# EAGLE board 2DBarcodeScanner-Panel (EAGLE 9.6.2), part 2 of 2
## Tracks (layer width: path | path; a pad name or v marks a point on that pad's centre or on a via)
3.3V  (via drill 0.38)
  Top 0.203: J4.3 23.37,16.38 29.34,22.35 32.3,22.35 J3.11 32.37,22.35 v34.04,22.35 | R7.2 43.14,24.64 v41.02,24.64 40.98,24.68 Q2.3 | 25.59,23.21 C2.1 | U1.5 25.59,23.21 | 25.59,23.21 25.59,22.41 v24.64,21.46
  Bottom 0.203: v24.64,21.46 25.53,22.35 v34.04,22.35 38.73,22.35 v41.02,24.64 | PWR.2 17.02,25.53 16.38,24.89 13.08,24.89 12.19,24 12.19,14.1 15.37,10.92 22.61,10.92 23.37,10.16 J4.3
3.3V1  (via drill 0.38)
  Top 0.203: J5.3 70.87,16.38 76.83,22.35 79.8,22.35 J6.11 79.87,22.35 v81.53,22.35 | R12.2 90.64,24.64 v88.52,24.64 88.48,24.68 Q4.3 | 73.09,23.21 C5.1 | U4.5 73.09,23.21 | 73.09,23.21 73.09,22.41 v72.14,21.46
  Bottom 0.203: v72.14,21.46 73.03,22.35 v81.53,22.35 86.23,22.35 v88.52,24.64 | PWR1.2 64.52,25.53 63.88,24.89 60.58,24.89 59.69,24 59.69,14.1 62.86,10.92 70.1,10.92 70.87,10.16 J5.3
3.3V2  (via drill 0.38)
  Top 0.203: J8.3 23.37,42.29 29.34,48.26 32.3,48.26 J9.11 32.37,48.26 v34.04,48.26 | R21.2 43.14,50.55 v41.02,50.55 40.98,50.59 Q6.3 | 25.59,49.12 C8.1 | U6.5 25.59,49.12 | 25.59,49.12 25.59,48.32 v24.64,47.37
  Bottom 0.203: v24.64,47.37 25.53,48.26 v34.04,48.26 38.73,48.26 v41.02,50.55 | PWR2.2 17.02,51.43 16.38,50.8 13.08,50.8 12.19,49.91 12.19,40 15.37,36.83 22.61,36.83 23.37,36.07 J8.3
3.3V3  (via drill 0.38)
  Top 0.203: J11.3 70.87,42.29 76.83,48.26 79.8,48.26 J12.11 79.87,48.26 v81.53,48.26 | R30.2 90.64,50.55 v88.52,50.55 88.48,50.59 Q8.3 | 73.09,49.12 C11.1 | U8.5 73.09,49.12 | 73.09,49.12 73.09,48.32 v72.14,47.37
  Bottom 0.203: v72.14,47.37 73.03,48.26 v81.53,48.26 86.23,48.26 v88.52,50.55 | PWR3.2 64.52,51.43 63.88,50.8 60.58,50.8 59.69,49.91 59.69,40 62.86,36.83 70.1,36.83 70.87,36.07 J11.3
3.3V4  (via drill 0.38)
  Top 0.203: J14.3 23.37,68.2 29.34,74.17 32.3,74.17 J15.11 32.37,74.17 v34.04,74.17 | R39.2 43.14,76.45 v41.02,76.45 40.98,76.5 Q10.3 | 25.59,75.03 C14.1 | U10.5 25.59,75.03 | 25.59,75.03 25.59,74.23 v24.64,73.28
  Bottom 0.203: v24.64,73.28 25.53,74.17 v34.04,74.17 38.73,74.17 v41.02,76.45 | PWR4.2 17.02,77.34 16.38,76.71 13.08,76.71 12.19,75.82 12.19,65.91 15.37,62.74 22.61,62.74 23.37,61.98 J14.3
3.3V5  (via drill 0.38)
  Top 0.203: J17.3 70.87,68.2 76.83,74.17 79.8,74.17 J18.11 79.87,74.17 v81.53,74.17 | R48.2 90.64,76.45 v88.52,76.45 88.48,76.5 Q12.3 | 73.09,75.03 C17.1 | U12.5 73.09,75.03 | 73.09,75.03 73.09,74.23 v72.14,73.28
  Bottom 0.203: v72.14,73.28 73.03,74.17 v81.53,74.17 86.23,74.17 v88.52,76.45 | PWR5.2 64.52,77.34 63.88,76.71 60.58,76.71 59.69,75.82 59.69,65.91 62.86,62.74 70.1,62.74 70.87,61.98 J17.3
3.3V6  (via drill 0.38)
  Top 0.203: J20.3 23.37,94.11 29.34,100.08 32.3,100.08 J21.11 32.37,100.08 v34.04,100.08 | R57.2 43.14,102.36 v41.02,102.36 40.98,102.41 Q14.3 | 25.59,100.94 C20.1 | U14.5 25.59,100.94 | 25.59,100.94 25.59,100.14 v24.64,99.19
  Bottom 0.203: v24.64,99.19 25.53,100.08 v34.04,100.08 38.73,100.08 v41.02,102.36 | PWR6.2 17.02,103.25 16.38,102.62 13.08,102.62 12.19,101.73 12.19,91.82 15.37,88.65 22.61,88.65 23.37,87.88 J20.3
3.3V7  (via drill 0.38)
  Top 0.203: J23.3 70.87,94.11 76.83,100.08 79.8,100.08 J24.11 79.87,100.08 v81.53,100.08 | R66.2 90.64,102.36 v88.52,102.36 88.48,102.41 Q16.3 | 73.09,100.94 C23.1 | U16.5 73.09,100.94 | 73.09,100.94 73.09,100.14 v72.14,99.19
  Bottom 0.203: v72.14,99.19 73.03,100.08 v81.53,100.08 86.23,100.08 v88.52,102.36 | PWR7.2 64.52,103.25 63.88,102.62 60.58,102.62 59.69,101.73 59.69,91.82 62.86,88.65 70.1,88.65 70.87,87.88 J23.3
5V  (via drill 0.38)
  Top 0.178: 25.62,27.3 U1.1
  Top 0.203: J2.VBUS1 15.5,22.1 v17.02,22.1 | v17.02,17.02 15.5,17.02 J2.VBUS2 | v25.53,30.1 25.49,30.06 C1.1 25.62,28.83 25.62,27.3 25.62,26.25 25.27,25.91 24,25.91 23.69,26.22 U1.3
  Bottom 0.203: v17.02,22.1 v17.02,17.02 20.83,17.02 23.37,19.56 23.37,27.94 v25.53,30.1
5V1  (via drill 0.38)
  Top 0.178: 73.12,27.3 U4.1
  Top 0.203: J1.VBUS1 63,22.1 v64.52,22.1 | v64.52,17.02 63,17.02 J1.VBUS2 | v73.03,30.1 72.99,30.06 C4.1 73.12,28.83 73.12,27.3 73.12,26.25 72.77,25.91 71.5,25.91 71.19,26.22 U4.3
  Bottom 0.203: v64.52,22.1 v64.52,17.02 68.33,17.02 70.87,19.56 70.87,27.94 v73.03,30.1
5V2  (via drill 0.38)
  Top 0.178: 25.62,53.21 U6.1
  Top 0.203: J7.VBUS1 15.5,48.01 v17.02,48.01 | v17.02,42.93 15.5,42.93 J7.VBUS2 | v25.53,56.01 25.49,55.97 C7.1 25.62,54.73 25.62,53.21 25.62,52.16 25.27,51.82 24,51.82 23.69,52.13 U6.3
  Bottom 0.203: v17.02,48.01 v17.02,42.93 20.83,42.93 23.37,45.47 23.37,53.85 v25.53,56.01
5V3  (via drill 0.38)
  Top 0.178: 73.12,53.21 U8.1
  Top 0.203: J10.VBUS1 63,48.01 v64.52,48.01 | v64.52,42.93 63,42.93 J10.VBUS2 | v73.03,56.01 72.99,55.97 C10.1 73.12,54.73 73.12,53.21 73.12,52.16 72.77,51.82 71.5,51.82 71.19,52.13 U8.3
  Bottom 0.203: v64.52,48.01 v64.52,42.93 68.33,42.93 70.87,45.47 70.87,53.85 v73.03,56.01
5V4  (via drill 0.38)
  Top 0.178: 25.62,79.12 U10.1
  Top 0.203: J13.VBUS1 15.5,73.91 v17.02,73.91 | v17.02,68.83 15.5,68.83 J13.VBUS2 | v25.53,81.92 25.49,81.88 C13.1 25.62,80.64 25.62,79.12 25.62,78.07 25.27,77.72 24,77.72 23.69,78.04 U10.3
  Bottom 0.203: v17.02,73.91 v17.02,68.83 20.83,68.83 23.37,71.37 23.37,79.76 v25.53,81.92
5V5  (via drill 0.38)
  Top 0.178: 73.12,79.12 U12.1
  Top 0.203: J16.VBUS1 63,73.91 v64.52,73.91 | v64.52,68.83 63,68.83 J16.VBUS2 | v73.03,81.92 72.99,81.88 C16.1 73.12,80.64 73.12,79.12 73.12,78.07 72.77,77.72 71.5,77.72 71.19,78.04 U12.3
  Bottom 0.203: v64.52,73.91 v64.52,68.83 68.33,68.83 70.87,71.37 70.87,79.76 v73.03,81.92
5V6  (via drill 0.38)
  Top 0.178: 25.62,105.03 U14.1
  Top 0.203: J19.VBUS1 15.5,99.82 v17.02,99.82 | v17.02,94.74 15.5,94.74 J19.VBUS2 | v25.53,107.82 25.49,107.78 C19.1 25.62,106.55 25.62,105.03 25.62,103.98 25.27,103.63 24,103.63 23.69,103.95 U14.3
  Bottom 0.203: v17.02,99.82 v17.02,94.74 20.83,94.74 23.37,97.28 23.37,105.66 v25.53,107.82
5V7  (via drill 0.38)
  Top 0.178: 73.12,105.03 U16.1
  Top 0.203: J22.VBUS1 63,99.82 v64.52,99.82 | v64.52,94.74 63,94.74 J22.VBUS2 | v73.03,107.82 72.99,107.78 C22.1 73.12,106.55 73.12,105.03 73.12,103.98 72.77,103.63 71.5,103.63 71.19,103.95 U16.3
  Bottom 0.203: v64.52,99.82 v64.52,94.74 68.33,94.74 70.87,97.28 70.87,105.66 v73.03,107.82
!SCAN_TRIGGER!  (via drill 0.38)
  Top 0.203: v35.31,24.64 S2.3 35.31,20.95 25.91,11.56 J4.2 | C3.1 35.27,27.43 v35.31,27.39 J3.1
  Bottom 0.203: v35.31,24.64 v35.31,27.39
!SCAN_TRIGGER!1  (via drill 0.38)
  Top 0.203: v82.8,24.64 S1.3 82.8,20.95 73.41,11.56 J5.2 | C6.1 82.77,27.43 v82.8,27.39 J6.1
  Bottom 0.203: v82.8,24.64 v82.8,27.39
!SCAN_TRIGGER!2  (via drill 0.38)
  Top 0.203: v35.31,50.55 S3.3 35.31,46.86 25.91,37.46 J8.2 | C9.1 35.27,53.33 v35.31,53.3 J9.1
  Bottom 0.203: v35.31,50.55 v35.31,53.3
!SCAN_TRIGGER!3  (via drill 0.38)
  Top 0.203: v82.8,50.55 S4.3 82.8,46.86 73.41,37.46 J11.2 | C12.1 82.77,53.33 v82.8,53.3 J12.1
  Bottom 0.203: v82.8,50.55 v82.8,53.3
!SCAN_TRIGGER!4  (via drill 0.38)
  Top 0.203: v35.31,76.45 S5.3 35.31,72.77 25.91,63.37 J14.2 | C15.1 35.27,79.24 v35.31,79.2 J15.1
  Bottom 0.203: v35.31,76.45 v35.31,79.2
!SCAN_TRIGGER!5  (via drill 0.38)
  Top 0.203: v82.8,76.45 S6.3 82.8,72.77 73.41,63.37 J17.2 | C18.1 82.77,79.24 v82.8,79.2 J18.1
  Bottom 0.203: v82.8,76.45 v82.8,79.2
!SCAN_TRIGGER!6  (via drill 0.38)
  Top 0.203: v35.31,102.36 S7.3 35.31,98.68 25.91,89.28 J20.2 | C21.1 35.27,105.15 v35.31,105.11 J21.1
  Bottom 0.203: v35.31,102.36 v35.31,105.11
!SCAN_TRIGGER!7  (via drill 0.38)
  Top 0.203: v82.8,102.36 S8.3 82.8,98.68 73.41,89.28 J23.2 | C24.1 82.77,105.15 v82.8,105.11 J24.1
  Bottom 0.203: v82.8,102.36 v82.8,105.11
BUZZER  (via drill 0.38)
  Top 0.203: v41.15,29.59 R9.1 | J3.4 31.01,25.89 v30.99,25.91
  Bottom 0.203: v30.99,25.91 30.99,28.45 32.13,29.59 v41.15,29.59
BUZZER1  (via drill 0.38)
  Top 0.203: v88.65,29.59 R14.1 | J6.4 78.51,25.89 v78.49,25.91
  Bottom 0.203: v78.49,25.91 78.49,28.45 79.63,29.59 v88.65,29.59
BUZZER2  (via drill 0.38)
  Top 0.203: v41.15,55.5 R23.1 | J9.4 31.01,51.8 v30.99,51.82
  Bottom 0.203: v30.99,51.82 30.99,54.36 32.13,55.5 v41.15,55.5
BUZZER3  (via drill 0.38)
  Top 0.203: v88.65,55.5 R32.1 | J12.4 78.51,51.8 v78.49,51.82
  Bottom 0.203: v78.49,51.82 78.49,54.36 79.63,55.5 v88.65,55.5
BUZZER4  (via drill 0.38)
  Top 0.203: v41.15,81.41 R41.1 | J15.4 31.01,77.7 v30.99,77.72
  Bottom 0.203: v30.99,77.72 30.99,80.26 32.13,81.41 v41.15,81.41
BUZZER5  (via drill 0.38)
  Top 0.203: v88.65,81.41 R50.1 | J18.4 78.51,77.7 v78.49,77.72
  Bottom 0.203: v78.49,77.72 78.49,80.26 79.63,81.41 v88.65,81.41
BUZZER6  (via drill 0.38)
  Top 0.203: v41.15,107.31 R59.1 | J21.4 31.01,103.61 v30.99,103.63
  Bottom 0.203: v30.99,103.63 30.99,106.17 32.13,107.31 v41.15,107.31
BUZZER7  (via drill 0.38)
  Top 0.203: v88.65,107.31 R68.1 | J24.4 78.51,103.61 v78.49,103.63
  Bottom 0.203: v78.49,103.63 78.49,106.17 79.63,107.31 v88.65,107.31
CC1
  Top 0.178: J1.A5 63.19,20.81
  Top 0.203: 63.19,20.81 65.85,20.81 R6.2
CC2
  Top 0.203: J1.B5 66.23,17.81 R5.2
CC3
  Top 0.178: J2.A5 15.69,20.81
  Top 0.203: 15.69,20.81 18.36,20.81 R3.2
CC4
  Top 0.203: J2.B5 18.74,17.81 R2.2
CC5
  Top 0.178: J7.A5 15.69,46.72
  Top 0.203: 15.69,46.72 18.36,46.72 R20.2
CC6
  Top 0.203: J7.B5 18.74,43.72 R19.2
CC7
  Top 0.178: J10.A5 63.19,46.72
  Top 0.203: 63.19,46.72 65.85,46.72 R29.2
CC8
  Top 0.203: J10.B5 66.23,43.72 R28.2
CC9
  Top 0.178: J13.A5 15.69,72.62
  Top 0.203: 15.69,72.62 18.36,72.62 R38.2
CC10
  Top 0.203: J13.B5 18.74,69.62 R37.2
CC11
  Top 0.178: J16.A5 63.19,72.62
  Top 0.203: 63.19,72.62 65.85,72.62 R47.2
CC12
  Top 0.203: J16.B5 66.23,69.62 R46.2
CC13
  Top 0.178: J19.A5 15.69,98.53
  Top 0.203: 15.69,98.53 18.36,98.53 R56.2
CC14
  Top 0.203: J19.B5 18.74,95.53 R55.2
CC15
  Top 0.178: J22.A5 63.19,98.53
  Top 0.203: 63.19,98.53 65.85,98.53 R65.2
CC16
  Top 0.203: J22.B5 66.23,95.53 R64.2
GND  (via drill 0.38)  (25 unrouted)
  Top 0.203: C1.2 24.64,28.11 U1.2 | C2.2 24.64,23.96 v24.64,24.64 | J3.10 33.43,22.89 v34.04,23.5
  other vias: 14.48,25.91 13.21,25.91 19.56,24.64 10.67,20.83 10.67,18.29 28.57,20.19 34.04,24.64 28.45,28.45 28.45,27.18 28.45,25.91 17.02,14.48
  pour Top (isolate 0.305): 9.4,6.86 53.85,6.86 53.85,32.26 9.4,32.26
  pour Bottom (isolate 0.305): 9.4,32.26 9.4,6.86 53.85,6.86 53.85,32.26
GND1  (via drill 0.38)  (25 unrouted)
  Top 0.203: C4.2 72.14,28.11 U4.2 | C5.2 72.14,23.96 v72.14,24.64 | J6.10 80.93,22.89 v81.53,23.5
  other vias: 61.98,25.91 60.71,25.91 67.06,24.64 58.17,20.83 58.17,18.29 76.07,20.19 81.53,24.64 75.95,28.45 75.95,27.18 75.95,25.91 64.52,14.48
  pour Top (isolate 0.305): 56.9,6.86 101.35,6.86 101.35,32.26 56.9,32.26
  pour Bottom (isolate 0.305): 56.9,32.26 56.9,6.86 101.35,6.86 101.35,32.26
GND2  (via drill 0.38)  (25 unrouted)
  Top 0.203: C7.2 24.64,54.01 U6.2 | C8.2 24.64,49.87 v24.64,50.55 | J9.10 33.43,48.8 v34.04,49.4
  other vias: 14.48,51.82 13.21,51.82 19.56,50.55 10.67,46.74 10.67,44.2 28.57,46.1 34.04,50.55 28.45,54.36 28.45,53.09 28.45,51.82 17.02,40.39
  pour Top (isolate 0.305): 9.4,32.77 53.85,32.77 53.85,58.17 9.4,58.17
  pour Bottom (isolate 0.305): 9.4,58.17 9.4,32.77 53.85,32.77 53.85,58.17
GND3  (via drill 0.38)  (25 unrouted)
  Top 0.203: C10.2 72.14,54.01 U8.2 | C11.2 72.14,49.87 v72.14,50.55 | J12.10 80.93,48.8 v81.53,49.4
  other vias: 61.98,51.82 60.71,51.82 67.06,50.55 58.17,46.74 58.17,44.2 76.07,46.1 81.53,50.55 75.95,54.36 75.95,53.09 75.95,51.82 64.52,40.39
  pour Top (isolate 0.305): 56.9,32.77 101.35,32.77 101.35,58.17 56.9,58.17
  pour Bottom (isolate 0.305): 56.9,58.17 56.9,32.77 101.35,32.77 101.35,58.17
GND4  (via drill 0.38)  (25 unrouted)
  Top 0.203: C13.2 24.64,79.92 U10.2 | C14.2 24.64,75.78 v24.64,76.45 | J15.10 33.43,74.7 v34.04,75.31
  other vias: 14.48,77.72 13.21,77.72 19.56,76.45 10.67,72.64 10.67,70.1 28.57,72.01 34.04,76.45 28.45,80.26 28.45,78.99 28.45,77.72 17.02,66.29
  pour Top (isolate 0.305): 9.4,58.67 53.85,58.67 53.85,84.07 9.4,84.07
  pour Bottom (isolate 0.305): 9.4,84.07 9.4,58.67 53.85,58.67 53.85,84.07
GND5  (via drill 0.38)  (25 unrouted)
  Top 0.203: C16.2 72.14,79.92 U12.2 | C17.2 72.14,75.78 v72.14,76.45 | J18.10 80.93,74.7 v81.53,75.31
  other vias: 61.98,77.72 60.71,77.72 67.06,76.45 58.17,72.64 58.17,70.1 76.07,72.01 81.53,76.45 75.95,80.26 75.95,78.99 75.95,77.72 64.52,66.29
  pour Top (isolate 0.305): 56.9,58.67 101.35,58.67 101.35,84.07 56.9,84.07
  pour Bottom (isolate 0.305): 56.9,84.07 56.9,58.67 101.35,58.67 101.35,84.07
GND6  (via drill 0.38)  (25 unrouted)
  Top 0.203: C19.2 24.64,105.83 U14.2 | C20.2 24.64,101.69 v24.64,102.36 | J21.10 33.43,100.61 v34.04,101.22
  other vias: 14.48,103.63 13.21,103.63 19.56,102.36 10.67,98.55 10.67,96.01 28.57,97.92 34.04,102.36 28.45,106.17 28.45,104.9 28.45,103.63 17.02,92.2
  pour Top (isolate 0.305): 9.4,84.58 53.85,84.58 53.85,109.98 9.4,109.98
  pour Bottom (isolate 0.305): 9.4,109.98 9.4,84.58 53.85,84.58 53.85,109.98
GND7  (via drill 0.38)  (25 unrouted)
  Top 0.203: C22.2 72.14,105.83 U16.2 | C23.2 72.14,101.69 v72.14,102.36 | J24.10 80.93,100.61 v81.53,101.22
  other vias: 61.98,103.63 60.71,103.63 67.06,102.36 58.17,98.55 58.17,96.01 76.07,97.92 81.53,102.36 75.95,106.17 75.95,104.9 75.95,103.63 64.52,92.2
  pour Top (isolate 0.305): 56.9,84.58 101.35,84.58 101.35,109.98 56.9,109.98
  pour Bottom (isolate 0.305): 56.9,109.98 56.9,84.58 101.35,84.58 101.35,109.98
N$1  (via drill 0.38)
  Top 0.203: R7.1 43.18,21.46 v43.05,21.34
  Bottom 0.203: v43.05,21.34 42.55,20.83 35.67,20.83 35.17,20.32 BUZZ.2
N$2
  Top 0.178: Q1.3 47.12,27.13
  Top 0.203: 47.12,16.12 48.77,14.48 LS1.-
  Top 0.254: 47.12,27.13 47.12,16.12
N$3  (via drill 0.38)
  Top 0.203: v39.88,14.48 LS1.+
  Bottom 0.203: BUZZ.1 38.48,19.43 39.88,18.03 v39.88,14.48
N$4
  Top 0.203: Q2.2 38.84,26.19 38.84,24.87 37.34,23.37 37.34,10.67 36.07,9.4 R1.2
N$5
  Top 0.203: R8.2 43.28,28.13 Q1.1 44.92,28.18 R9.2
N$6  (via drill 0.38)
  Top 0.203: R4.1 v17.02,29.34
  Bottom 0.203: v17.02,29.34 PWR.1
N$7
  Top 0.203: R10.2 37.38,28.07 R11.2 37.44,28.13 Q2.1
N$8  (via drill 0.38)
  Top 0.203: v35.31,11.43 35.18,11.3 D2.A
  Bottom 0.203: PWR_LED.1 36.32,16.52 36.32,11.81 35.94,11.43 v35.31,11.43
N$9
  Top 0.203: D1.A 17.05,26.3 R4.2
N$10
  Top 0.178: Q3.3 94.62,27.13
  Top 0.203: 94.62,16.12 96.27,14.48 LS2.-
  Top 0.254: 94.62,27.13 94.62,16.12
N$11
  Top 0.203: R13.2 90.78,28.13 Q3.1 92.42,28.18 R14.2
N$12
  Top 0.203: Q4.2 86.33,26.19 86.33,24.87 84.84,23.37 84.84,10.67 83.57,9.4 R18.2
N$13
  Top 0.203: R15.2 84.88,28.07 R16.2 84.94,28.13 Q4.1
N$14  (via drill 0.38)
  Top 0.203: v82.8,11.43 82.68,11.3 D4.A
  Bottom 0.203: PWR_LED1.1 83.82,16.52 83.82,11.81 83.44,11.43 v82.8,11.43
N$15  (via drill 0.38)
  Top 0.203: R12.1 90.68,21.46 v90.55,21.34
  Bottom 0.203: v90.55,21.34 90.04,20.83 83.17,20.83 82.66,20.32 BUZZ1.2
N$16  (via drill 0.38)
  Top 0.203: v87.38,14.48 LS2.+
  Bottom 0.203: BUZZ1.1 85.98,19.43 87.38,18.03 v87.38,14.48
N$17  (via drill 0.38)
  Top 0.203: R17.1 v64.52,29.34
  Bottom 0.203: v64.52,29.34 PWR1.1
N$18
  Top 0.203: D3.A 64.54,26.3 R17.2
N$19
  Top 0.178: Q5.3 47.12,53.04
  Top 0.203: 47.12,42.03 48.77,40.39 LS3.-
  Top 0.254: 47.12,53.04 47.12,42.03
N$20
  Top 0.203: R22.2 43.28,54.04 Q5.1 44.92,54.09 R23.2
N$21
  Top 0.203: Q6.2 38.84,52.09 38.84,50.77 37.34,49.28 37.34,36.58 36.07,35.31 R27.2
N$22
  Top 0.203: R24.2 37.38,53.97 R25.2 37.44,54.04 Q6.1
N$23  (via drill 0.38)
  Top 0.203: v35.31,37.34 35.18,37.21 D6.A
  Bottom 0.203: PWR_LED2.1 36.32,42.43 36.32,37.72 35.94,37.34 v35.31,37.34
N$24  (via drill 0.38)
  Top 0.203: R21.1 43.18,47.37 v43.05,47.24
  Bottom 0.203: v43.05,47.24 42.55,46.74 35.67,46.74 35.17,46.23 BUZZ2.2
N$25  (via drill 0.38)
  Top 0.203: v39.88,40.39 LS3.+
  Bottom 0.203: BUZZ2.1 38.48,45.34 39.88,43.94 v39.88,40.39
N$26  (via drill 0.38)
  Top 0.203: R26.1 v17.02,55.24
  Bottom 0.203: v17.02,55.24 PWR2.1
N$27
  Top 0.203: D5.A 17.05,52.21 R26.2
N$28
  Top 0.178: Q7.3 94.62,53.04
  Top 0.203: 94.62,42.03 96.27,40.39 LS4.-
  Top 0.254: 94.62,53.04 94.62,42.03
N$29
  Top 0.203: R31.2 90.78,54.04 Q7.1 92.42,54.09 R32.2
N$30
  Top 0.203: Q8.2 86.33,52.09 86.33,50.77 84.84,49.28 84.84,36.58 83.57,35.31 R36.2
N$31
  Top 0.203: R33.2 84.88,53.97 R34.2 84.94,54.04 Q8.1
N$32  (via drill 0.38)
  Top 0.203: v82.8,37.34 82.68,37.21 D8.A
  Bottom 0.203: PWR_LED3.1 83.82,42.43 83.82,37.72 83.44,37.34 v82.8,37.34
N$33  (via drill 0.38)
  Top 0.203: R30.1 90.68,47.37 v90.55,47.24
  Bottom 0.203: v90.55,47.24 90.04,46.74 83.17,46.74 82.66,46.23 BUZZ3.2
N$34  (via drill 0.38)
  Top 0.203: v87.38,40.39 LS4.+
  Bottom 0.203: BUZZ3.1 85.98,45.34 87.38,43.94 v87.38,40.39
N$35  (via drill 0.38)
  Top 0.203: R35.1 v64.52,55.24
  Bottom 0.203: v64.52,55.24 PWR3.1
N$36
  Top 0.203: D7.A 64.54,52.21 R35.2
N$37
  Top 0.178: Q9.3 47.12,78.94
  Top 0.203: 47.12,67.94 48.77,66.29 LS5.-
  Top 0.254: 47.12,78.94 47.12,67.94
N$38
  Top 0.203: R40.2 43.28,79.94 Q9.1 44.92,80 R41.2
N$39
  Top 0.203: Q10.2 38.84,78 38.84,76.68 37.34,75.18 37.34,62.48 36.07,61.21 R45.2
N$40
  Top 0.203: R42.2 37.38,79.88 R43.2 37.44,79.94 Q10.1
N$41  (via drill 0.38)
  Top 0.203: v35.31,63.25 35.18,63.12 D10.A
  Bottom 0.203: PWR_LED4.1 36.32,68.34 36.32,63.63 35.94,63.25 v35.31,63.25
N$42  (via drill 0.38)
  Top 0.203: R39.1 43.18,73.28 v43.05,73.15
  Bottom 0.203: v43.05,73.15 42.55,72.64 35.67,72.64 35.17,72.14 BUZZ4.2
N$43  (via drill 0.38)
  Top 0.203: v39.88,66.29 LS5.+
  Bottom 0.203: BUZZ4.1 38.48,71.25 39.88,69.85 v39.88,66.29
N$44  (via drill 0.38)
  Top 0.203: R44.1 v17.02,81.15
  Bottom 0.203: v17.02,81.15 PWR4.1
N$45
  Top 0.203: D9.A 17.05,78.12 R44.2
N$46
  Top 0.178: Q11.3 94.62,78.94
  Top 0.203: 94.62,67.94 96.27,66.29 LS6.-
  Top 0.254: 94.62,78.94 94.62,67.94
N$47
  Top 0.203: R49.2 90.78,79.94 Q11.1 92.42,80 R50.2
N$48
  Top 0.203: Q12.2 86.33,78 86.33,76.68 84.84,75.18 84.84,62.48 83.57,61.21 R54.2
N$49
  Top 0.203: R51.2 84.88,79.88 R52.2 84.94,79.94 Q12.1
N$50  (via drill 0.38)
  Top 0.203: v82.8,63.25 82.68,63.12 D12.A
  Bottom 0.203: PWR_LED5.1 83.82,68.34 83.82,63.63 83.44,63.25 v82.8,63.25
N$51  (via drill 0.38)
  Top 0.203: R48.1 90.68,73.28 v90.55,73.15
  Bottom 0.203: v90.55,73.15 90.04,72.64 83.17,72.64 82.66,72.14 BUZZ5.2
N$52  (via drill 0.38)
  Top 0.203: v87.38,66.29 LS6.+
  Bottom 0.203: BUZZ5.1 85.98,71.25 87.38,69.85 v87.38,66.29
N$53  (via drill 0.38)
  Top 0.203: R53.1 v64.52,81.15
  Bottom 0.203: v64.52,81.15 PWR5.1
N$54
  Top 0.203: D11.A 64.54,78.12 R53.2
N$55
  Top 0.178: Q13.3 47.12,104.85
  Top 0.203: 47.12,93.85 48.77,92.2 LS7.-
  Top 0.254: 47.12,104.85 47.12,93.85
N$56
  Top 0.203: R58.2 43.28,105.85 Q13.1 44.92,105.91 R59.2
N$57
  Top 0.203: Q14.2 38.84,103.91 38.84,102.59 37.34,101.09 37.34,88.39 36.07,87.12 R63.2
N$58
  Top 0.203: R60.2 37.38,105.79 R61.2 37.44,105.85 Q14.1
N$59  (via drill 0.38)
  Top 0.203: v35.31,89.15 35.18,89.03 D14.A
  Bottom 0.203: PWR_LED6.1 36.32,94.25 36.32,89.54 35.94,89.15 v35.31,89.15
N$60  (via drill 0.38)
  Top 0.203: R57.1 43.18,99.19 v43.05,99.06
  Bottom 0.203: v43.05,99.06 42.55,98.55 35.67,98.55 35.17,98.04 BUZZ6.2
N$61  (via drill 0.38)
  Top 0.203: v39.88,92.2 LS7.+
  Bottom 0.203: BUZZ6.1 38.48,97.16 39.88,95.76 v39.88,92.2
N$62  (via drill 0.38)
  Top 0.203: R62.1 v17.02,107.06
  Bottom 0.203: v17.02,107.06 PWR6.1
N$63
  Top 0.203: D13.A 17.05,104.03 R62.2
N$64
  Top 0.178: Q15.3 94.62,104.85
  Top 0.203: 94.62,93.85 96.27,92.2 LS8.-
  Top 0.254: 94.62,104.85 94.62,93.85
N$65
  Top 0.203: R67.2 90.78,105.85 Q15.1 92.42,105.91 R68.2
N$66
  Top 0.203: Q16.2 86.33,103.91 86.33,102.59 84.84,101.09 84.84,88.39 83.57,87.12 R72.2
N$67
  Top 0.203: R69.2 84.88,105.79 R70.2 84.94,105.85 Q16.1
N$68  (via drill 0.38)
  Top 0.203: v82.8,89.15 82.68,89.03 D16.A
  Bottom 0.203: PWR_LED7.1 83.82,94.25 83.82,89.54 83.44,89.15 v82.8,89.15
N$69  (via drill 0.38)
  Top 0.203: R66.1 90.68,99.19 v90.55,99.06
  Bottom 0.203: v90.55,99.06 90.04,98.55 83.17,98.55 82.66,98.04 BUZZ7.2
N$70  (via drill 0.38)
  Top 0.203: v87.38,92.2 LS8.+
  Bottom 0.203: BUZZ7.1 85.98,97.16 87.38,95.76 v87.38,92.2
N$71  (via drill 0.38)
  Top 0.203: R71.1 v64.52,107.06
  Bottom 0.203: v64.52,107.06 PWR7.1
N$72
  Top 0.203: D15.A 64.54,104.03 R71.2
RXI
  Top 0.203: J3.9 32.27,23.32 29.64,23.32 20.83,14.51 J4.4
RXI1
  Top 0.203: J6.9 79.77,23.32 77.13,23.32 68.33,14.51 J5.4
RXI2
  Top 0.203: J9.9 32.27,49.22 29.64,49.22 20.83,40.42 J8.4
RXI3
  Top 0.203: J12.9 79.77,49.22 77.13,49.22 68.33,40.42 J11.4
RXI4
  Top 0.203: J15.9 32.27,75.13 29.64,75.13 20.83,66.33 J14.4
RXI5
  Top 0.203: J18.9 79.77,75.13 77.13,75.13 68.33,66.33 J17.4
RXI6
  Top 0.203: J21.9 32.27,101.04 29.64,101.04 20.83,92.23 J20.4
RXI7
  Top 0.203: J24.9 79.77,101.04 77.13,101.04 68.33,92.23 J23.4
STATUS_LED
  Top 0.203: R11.1 37.28,26.39 J3.3
STATUS_LED1
  Top 0.203: R16.1 84.78,26.39 J6.3
STATUS_LED2
  Top 0.203: R25.1 37.28,52.3 J9.3
STATUS_LED3
  Top 0.203: R34.1 84.78,52.3 J12.3
STATUS_LED4
  Top 0.203: R43.1 37.28,78.2 J15.3
STATUS_LED5
  Top 0.203: R52.1 84.78,78.2 J18.3
STATUS_LED6
  Top 0.203: R61.1 37.28,104.11 J21.3
STATUS_LED7
  Top 0.203: R70.1 84.78,104.11 J24.3
STATUS_OUT
  Top 0.203: R1.1 31.15,9.4 29.88,8.13 J4.1
  Bottom 0.203: PWR_LED.2 33.02,16.64 28.45,12.06 J4.1
STATUS_OUT1
  Top 0.203: R18.1 78.65,9.4 77.38,8.13 J5.1
  Bottom 0.203: PWR_LED1.2 80.52,16.64 75.95,12.06 J5.1
STATUS_OUT2
  Top 0.203: R27.1 31.15,35.31 29.88,34.04 J8.1
  Bottom 0.203: PWR_LED2.2 33.02,42.54 28.45,37.97 J8.1
STATUS_OUT3
  Top 0.203: R36.1 78.65,35.31 77.38,34.04 J11.1
  Bottom 0.203: PWR_LED3.2 80.52,42.54 75.95,37.97 J11.1
STATUS_OUT4
  Top 0.203: R45.1 31.15,61.21 29.88,59.94 J14.1
  Bottom 0.203: PWR_LED4.2 33.02,68.45 28.45,63.88 J14.1
STATUS_OUT5
  Top 0.203: R54.1 78.65,61.21 77.38,59.94 J17.1
  Bottom 0.203: PWR_LED5.2 80.52,68.45 75.95,63.88 J17.1
STATUS_OUT6
  Top 0.203: R63.1 31.15,87.12 29.88,85.85 J20.1
  Bottom 0.203: PWR_LED6.2 33.02,94.36 28.45,89.79 J20.1
STATUS_OUT7
  Top 0.203: R72.1 78.65,87.12 77.38,85.85 J23.1
  Bottom 0.203: PWR_LED7.2 80.52,94.36 75.95,89.79 J23.1
TXO
  Top 0.203: J4.5 18.29,12.54 29.63,23.89 J3.8
TXO1
  Top 0.203: J5.5 65.79,12.54 77.13,23.89 J6.8
TXO2
  Top 0.203: J8.5 18.29,38.45 29.63,49.8 J9.8
TXO3
  Top 0.203: J11.5 65.79,38.45 77.13,49.8 J12.8
TXO4
  Top 0.203: J14.5 18.29,64.36 29.63,75.7 J15.8
TXO5
  Top 0.203: J17.5 65.79,64.36 77.13,75.7 J18.8
TXO6
  Top 0.203: J20.5 18.29,90.27 29.63,101.61 J21.8
TXO7
  Top 0.203: J23.5 65.79,90.27 77.13,101.61 J24.8
USB_N  (via drill 0.38)
  Top 0.178: J2.B7 14.24,20.31 v13.46,21.08 | J2.A7 13.36,19.31 v13.33,19.28
  Top 0.203: J2.A7 15.47,19.25 18.99,19.25 20.36,17.88 22.96,17.88 29.47,24.39 J3.7
  Bottom 0.178: v13.46,21.08 14.1,20.45 14.1,20.04 v13.33,19.28
USB_N1  (via drill 0.38)
  Top 0.178: J1.B7 61.73,20.31 v60.96,21.08 | J1.A7 60.86,19.31 v60.83,19.28
  Top 0.203: J1.A7 62.97,19.25 66.49,19.25 67.85,17.88 70.46,17.88 76.97,24.39 J6.7
  Bottom 0.178: v60.96,21.08 61.59,20.45 61.59,20.04 v60.83,19.28
USB_N2  (via drill 0.38)
  Top 0.178: J7.B7 14.24,46.22 v13.46,46.99 | J7.A7 13.36,45.22 v13.33,45.19
  Top 0.203: J7.A7 15.47,45.15 18.99,45.15 20.36,43.79 22.96,43.79 29.47,50.3 J9.7
  Bottom 0.178: v13.46,46.99 14.1,46.35 14.1,45.95 v13.33,45.19
USB_N3  (via drill 0.38)
  Top 0.178: J10.B7 61.73,46.22 v60.96,46.99 | J10.A7 60.86,45.22 v60.83,45.19
  Top 0.203: J10.A7 62.97,45.15 66.49,45.15 67.85,43.79 70.46,43.79 76.97,50.3 J12.7
  Bottom 0.178: v60.96,46.99 61.59,46.35 61.59,45.95 v60.83,45.19
USB_N4  (via drill 0.38)
  Top 0.178: J13.B7 14.24,72.12 v13.46,72.9 | J13.A7 13.36,71.12 v13.33,71.09
  Top 0.203: J13.A7 15.47,71.06 18.99,71.06 20.36,69.7 22.96,69.7 29.47,76.2 J15.7
  Bottom 0.178: v13.46,72.9 14.1,72.26 14.1,71.86 v13.33,71.09
USB_N5  (via drill 0.38)
  Top 0.178: J16.B7 61.73,72.12 v60.96,72.9 | J16.A7 60.86,71.12 v60.83,71.09
  Top 0.203: J16.A7 62.97,71.06 66.49,71.06 67.85,69.7 70.46,69.7 76.97,76.2 J18.7
  Bottom 0.178: v60.96,72.9 61.59,72.26 61.59,71.86 v60.83,71.09
USB_N6  (via drill 0.38)
  Top 0.178: J19.B7 14.24,98.03 v13.46,98.81 | J19.A7 13.36,97.03 v13.33,97
  Top 0.203: J19.A7 15.47,96.97 18.99,96.97 20.36,95.61 22.96,95.61 29.47,102.11 J21.7
  Bottom 0.178: v13.46,98.81 14.1,98.17 14.1,97.77 v13.33,97
USB_N7  (via drill 0.38)
  Top 0.178: J22.B7 61.73,98.03 v60.96,98.81 | J22.A7 60.86,97.03 v60.83,97
  Top 0.203: J22.A7 62.97,96.97 66.49,96.97 67.85,95.61 70.46,95.61 76.97,102.11 J24.7
  Bottom 0.178: v60.96,98.81 61.59,98.17 61.59,97.77 v60.83,97
USB_P  (via drill 0.38)
  Top 0.178: J2.A6 13.9,19.81 13.46,20.24 v13.08,20.24 | J2.B6 13.83,18.81 13.33,18.31 v13.21,18.31
  Top 0.203: J2.A6 19.06,19.81 20.5,18.36 22.87,18.36 29.4,24.89 J3.6
  Bottom 0.178: v13.08,20.24 12.7,19.86 12.7,18.67 13.06,18.31 v13.21,18.31
USB_P1  (via drill 0.38)
  Top 0.178: J1.A6 61.4,19.81 60.96,20.24 v60.58,20.24 | J1.B6 61.33,18.81 60.83,18.31 v60.71,18.31
  Top 0.203: J1.A6 66.56,19.81 68,18.36 70.37,18.36 76.89,24.89 J6.6
  Bottom 0.178: v60.58,20.24 60.2,19.86 60.2,18.67 60.55,18.31 v60.71,18.31
USB_P2  (via drill 0.38)
  Top 0.178: J7.A6 13.9,45.72 13.46,46.15 v13.08,46.15 | J7.B6 13.83,44.72 13.33,44.22 v13.21,44.22
  Top 0.203: J7.A6 19.06,45.72 20.5,44.27 22.87,44.27 29.4,50.8 J9.6
  Bottom 0.178: v13.08,46.15 12.7,45.77 12.7,44.58 13.06,44.22 v13.21,44.22
USB_P3  (via drill 0.38)
  Top 0.178: J10.A6 61.4,45.72 60.96,46.15 v60.58,46.15 | J10.B6 61.33,44.72 60.83,44.22 v60.71,44.22
  Top 0.203: J10.A6 66.56,45.72 68,44.27 70.37,44.27 76.89,50.8 J12.6
  Bottom 0.178: v60.58,46.15 60.2,45.77 60.2,44.58 60.55,44.22 v60.71,44.22
USB_P4  (via drill 0.38)
  Top 0.178: J13.A6 13.9,71.62 13.46,72.06 v13.08,72.06 | J13.B6 13.83,70.62 13.33,70.13 v13.21,70.13
  Top 0.203: J13.A6 19.06,71.62 20.5,70.18 22.87,70.18 29.4,76.7 J15.6
  Bottom 0.178: v13.08,72.06 12.7,71.68 12.7,70.48 13.06,70.13 v13.21,70.13
USB_P5  (via drill 0.38)
  Top 0.178: J16.A6 61.4,71.62 60.96,72.06 v60.58,72.06 | J16.B6 61.33,70.62 60.83,70.13 v60.71,70.13
  Top 0.203: J16.A6 66.56,71.62 68,70.18 70.37,70.18 76.89,76.7 J18.6
  Bottom 0.178: v60.58,72.06 60.2,71.68 60.2,70.48 60.55,70.13 v60.71,70.13
USB_P6  (via drill 0.38)
  Top 0.178: J19.A6 13.9,97.53 13.46,97.97 v13.08,97.97 | J19.B6 13.83,96.53 13.33,96.04 v13.21,96.04
  Top 0.203: J19.A6 19.06,97.53 20.5,96.09 22.87,96.09 29.4,102.61 J21.6
  Bottom 0.178: v13.08,97.97 12.7,97.59 12.7,96.39 13.06,96.04 v13.21,96.04
USB_P7  (via drill 0.38)
  Top 0.178: J22.A6 61.4,97.53 60.96,97.97 v60.58,97.97 | J22.B6 61.33,96.53 60.83,96.04 v60.71,96.04
  Top 0.203: J22.A6 66.56,97.53 68,96.09 70.37,96.09 76.89,102.61 J24.6
  Bottom 0.178: v60.58,97.97 60.2,97.59 60.2,96.39 60.55,96.04 v60.71,96.04

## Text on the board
Bottom: v11 | v11 | v11 | v11 | v11 | v11 | v11 | v11
Dimension: Route Out | Route Out | Route Out | Route Out | Route Out | Route Out | Route Out | Route Out | Route Out | Route Out | Route Out | Route Out | Route Out | Route Out | Route Out | Route Out | Route Out | Route Out | Route Out | Route Out
Milling: v-score | v-score | v-score | v-score | v-score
